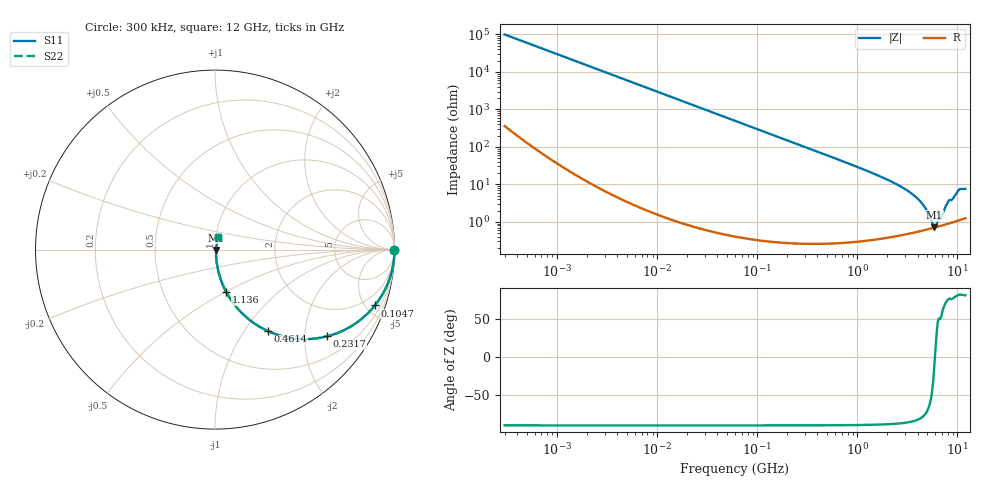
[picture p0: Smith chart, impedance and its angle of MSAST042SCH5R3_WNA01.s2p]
! MSAST042SCH5R3_WNA01  S-PARAMETER MODEL  ( General Type )
! Model Generated by TAIYO YUDEN Corporation (http://www.ty-top.com)
! Version 1.0
! TAIYO YUDEN Control No. 150820
! Copyright(c) 2015 TAIYO YUDEN CO.,LTD. All Rights Reserved.
! Product Description (link to TY-COMPAS)
! https://ds.yuden.co.jp/TYCOMPAS/or/detail?pn=MSAST042SCH5R3BWNA01&u=M
! Products Name : Multilayer Ceramic Capacitors
! Characteristics :
!  Capacitance : 5.3 pF , Rated Voltage : 25V , TCC : CH / C0H
!  Case Size : 0.4 x 0.2 / 0.016 x 0.008 [mm/inch] , Thickness : 0.2 / 0.008 [mm/inch]
!  (Conditions: Temperature = 25 degC , DC Bias Current/Voltage = 0A / 0V)
! External Node Assignments :
!  1  o---| |---o  2
! GND o---------o GND
! Frequency Range : 0.3MHz  -  12000MHz  [ 401 STEP ]
# MHz S RI R 50
! Freq[MHz].  S11 Real  S11 Imag  S21 Real  S21 Imag  S12 Real  S12 Imag  S22 Real  S22 Imag
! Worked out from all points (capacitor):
!   401 points, 300 kHz to 12 GHz, reference 50 ohm
!   read as one part in series: C = 5.31 pF near 316.3 kHz
!   lowest |Z| = 717 mohm at 5.869 GHz (marker M1)
!   series resonance near 5.957 GHz, so ESL is about 130 pH
!   S11 on the Smith chart (normalised r, x): 300 kHz: open; 104.7 MHz: 1.01, -5.72; 231.7 MHz: 1.01, -2.58; 461.4 MHz: 1.01, -1.29; 1.136 GHz: 1.01, -0.51; 12 GHz: 1.02, +0.15
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0.3  1 -0.001  4.61e-06 0.001  4.61e-06 0.001  1 -0.001
1.769972  1 -0.00591  3.99e-05 0.00591  3.99e-05 0.00591  1 -0.00591
10.44266  0.9988 -0.0348  0.00123 0.0348  0.00123 0.0348  0.9988 -0.0348
27.82928  0.9914 -0.0921  0.00861 0.0921  0.00861 0.0921  0.9914 -0.0921
60  0.9613 -0.1925  0.0387 0.1925  0.0387 0.1925  0.9613 -0.1925
104.6549  0.8909 -0.3112  0.1091 0.3112  0.1091 0.3112  0.8909 -0.3112
155.7172  0.7867 -0.4089  0.2133 0.4089  0.2133 0.4089  0.7867 -0.4089
231.6935  0.6247 -0.4832  0.3753 0.4832  0.3753 0.4832  0.6247 -0.4832
353.9943  0.4158 -0.4913  0.5842 0.4913  0.5842 0.4913  0.4158 -0.4913
461.3684  0.2948 -0.454  0.7052 0.454  0.7052 0.454  0.2948 -0.454
704.9044  0.151 -0.3548  0.849 0.3548  0.849 0.3548  0.151 -0.3548
1135.593  0.0632 -0.2374  0.9368 0.2374  0.9368 0.2374  0.0632 -0.2374
2088.533  0.0192 -0.123  0.9808 0.123  0.9808 0.123  0.0192 -0.123
3107.553  0.0095 -0.0693  0.9905 0.0693  0.9905 0.0693  0.0095 -0.0693
4050.141  0.007 -0.0394  0.993 0.0394  0.993 0.0394  0.007 -0.0394
4747.894  0.00654 -0.0229  0.9935 0.0229  0.9935 0.0229  0.00654 -0.0229
5565.855  0.00674 -0.00694  0.9933 0.00694  0.9933 0.00694  0.00674 -0.00694
5868.704  0.00695 -0.00155  0.993 0.00155  0.993 0.00155  0.00695 -0.00155
6524.734  0.00758 0.00887  0.9924 -0.00887  0.9924 -0.00887  0.00758 0.00887
8064.993  0.00989 0.0327  0.9901 -0.0327  0.9901 -0.0327  0.00989 0.0327
10511.28  0.0162 0.0721  0.9838 -0.0721  0.9838 -0.0721  0.0162 0.0721
12000  0.0176 0.0722  0.9824 -0.0722  0.9824 -0.0722  0.0176 0.0722
